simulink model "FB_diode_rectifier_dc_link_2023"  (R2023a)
settings: Solver=VariableStepAuto  StartTime=0.0  StopTime=0.1  MaxStep=1e-5  RelTol=1e-3
libraries: spsDiodeLib x4, spsCurrentMeasurementLib x2, spsSeriesRLCBranchLib x2, spsVoltageMeasurementLib x2, spsACVoltageSourceLib x1, spsGroundLib x1, spsPowerLib x1, spspowerguiLib x1

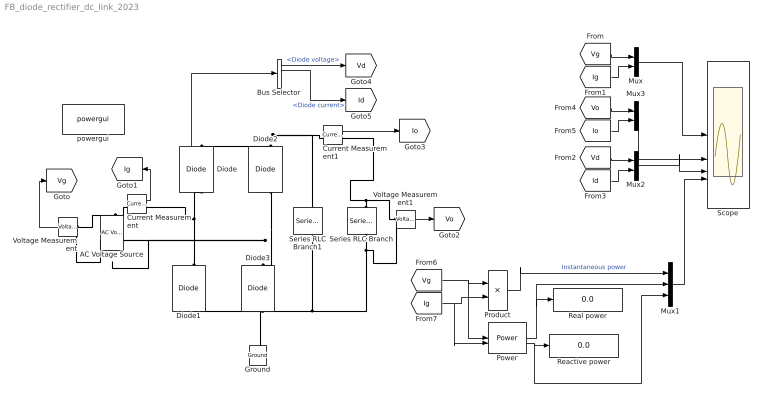
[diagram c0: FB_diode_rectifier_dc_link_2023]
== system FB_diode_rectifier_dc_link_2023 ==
  AC Voltage Source : spsACVoltageSourceLib/AC Voltage Source  Amplitude=220*sqrt(2)  Phase=0  Frequency=60  SampleTime=0  Measurements=None  BusType=swing  Pref=10e3  Qref=0  Qmin=-inf  Qmax=+inf
  Bus Selector : BusSelector  OutputSignals=Diode voltage,Diode current
  Current Measurement : spsCurrentMeasurementLib/Current Measurement  PhasorSimulation=off  OutputType=Complex  PSBequivalent=0
  Current Measurement1 : spsCurrentMeasurementLib/Current Measurement  PhasorSimulation=off  OutputType=Complex  PSBequivalent=0
  Diode{,1..3} (4 alike) : spsDiodeLib/Diode  Ron=0.001  Lon=0  Vf=0.8  IC=0  UseSnubber=0  Rs=500  Cs=250e-9  Measurements=on
  Ground : spsGroundLib/Ground  LConnTagsString=a
  Mux : Mux  Inputs=2
  Mux1 : Mux  Inputs=3
  Mux2 : Mux  Inputs=2
  Mux3 : Mux  Inputs=2
  Power : spsPowerLib/Power  Freq=60  Vinit=[1, 0]  Iinit=[1, 0]  Ts=0
  Product : Product
  Reactive power : Display
  Real power : Display
  Scope : Scope  NumInputPorts=4
  Series RLC Branch : spsSeriesRLCBranchLib/Series RLC Branch  LConnTagsString=__new0  RConnTagsString=__new0  BranchType=R  Resistance=50  Inductance=1e-3  SetiL0=off  InitialCurrent=0  Capacitance=1e-6  Setx0=off  InitialVoltage=0  Measurements=None
  Series RLC Branch1 : spsSeriesRLCBranchLib/Series RLC Branch  LConnTagsString=__new0  RConnTagsString=__new0  BranchType=C  Resistance=5  Inductance=1e-3  SetiL0=off  InitialCurrent=0  Capacitance=4700e-6  Setx0=on  InitialVoltage=311  Measurements=None
  Voltage Measurement : spsVoltageMeasurementLib/Voltage Measurement  PhasorSimulation=off  OutputType=Complex  PSBequivalent=0
  Voltage Measurement1 : spsVoltageMeasurementLib/Voltage Measurement  PhasorSimulation=off  OutputType=Complex  PSBequivalent=0
  powergui : spspowerguiLib/powergui  Priority=1  SimulationMode=Continuous  SampleTime=50e-6  frequency=60  Iterations=50  frequencyindice=60  Pbase=100e6  ErrMax=1e-4  UnitsV=kV  UnitsW=MW  buscounter=0  FunctionMessages=off  echomessages=off  EnableUseOfTLC=off  CurrentSourceSwitches=off  DisableSnubberDevices=off  DisableRonSwitches=off  DisableVfSwitches=off  DisplayEquations=off  AutomaticDiscreteSolvers=off  SolverType=Tustin/Backward Euler (TBE)  Interpol=off  ExternalGateDelay=off  methode=off  Ts=100  x0status=blocks  SPID=on  SwTol=0  HookPort=off  NonlinearTolerance=1e-4  nMaxIteration=100  ContinueOnMaxIteration=off  RestoreLinks=warning  ResistiveCurrentMeasurement=off  Frange=[0:2:500]  Ylog=off  Xlog=on  ShowGrid=off  save=off  variable=ZData  structure=0  ZoomFFT=off  StartTime=0.0  cycles=1  DisplayStyle=1  fundamental=60  FreqAxis=off  MaxFrequency=1000  frequencyindicesteady=1  RmsSteady=1  display=off
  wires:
  Power/1 -> Mux1/2, Real power/1
  Power/2 -> Mux1/3, Reactive power/1
  Product/1 -> Mux1/1  "Instantaneous power"
  Voltage Measurement/1 -> [Vg]
  Current Measurement/1 -> [Ig]
  Voltage Measurement1/1 -> [Vo]
  Current Measurement1/1 -> [Io]
  Diode/1 -> Bus Selector/1
  [Vg] -> Mux/1
  [Ig] -> Mux/2
  Mux/1 -> Scope/1
  Bus Selector/1 -> [Vd]  "<Diode voltage>"
  Bus Selector/2 -> [Id]  "<Diode current>"
  [Vd] -> Mux2/1
  [Id] -> Mux2/2
  Mux2/1 -> Scope/3
  Mux3/1 -> Scope/2
  [Vo] -> Mux3/1
  [Io] -> Mux3/2
  Mux1/1 -> Scope/4
  [Vg] -> Power/1, Product/1
  [Ig] -> Power/2, Product/2
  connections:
  Diode1/RConn1 -- Current Measurement/RConn1 -- Diode/LConn1
  Diode2/LConn1 -- Voltage Measurement/LConn2 -- AC Voltage Source/LConn1 -- Diode3/RConn1
  AC Voltage Source/RConn1 -- Current Measurement/LConn1 -- Voltage Measurement/LConn1
  Series RLC Branch/LConn1 -- Voltage Measurement1/LConn1 -- Current Measurement1/RConn1
  Series RLC Branch/RConn1 -- Voltage Measurement1/LConn2 -- Series RLC Branch1/RConn1 -- Ground/LConn1 -- Diode1/LConn1 -- Diode3/LConn1
  Diode/RConn1 -- Series RLC Branch1/LConn1 -- Current Measurement1/LConn1 -- Diode2/RConn1
